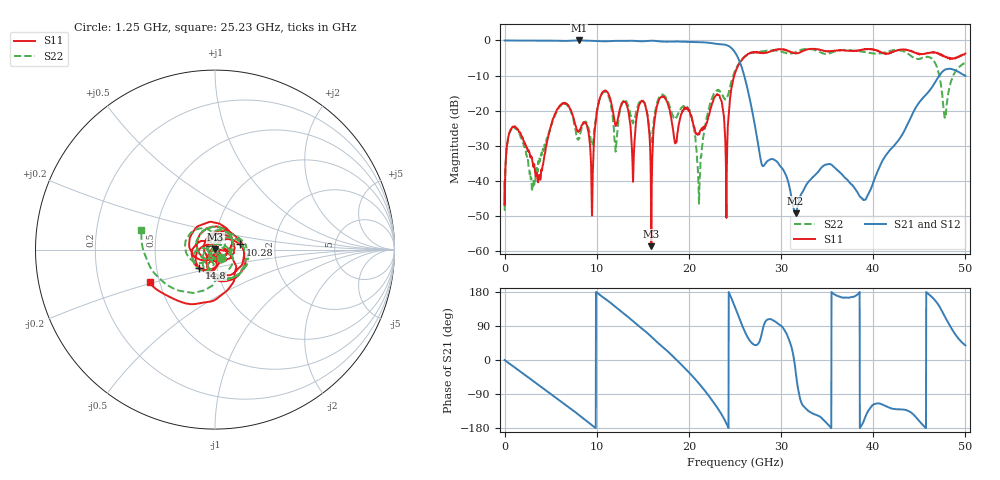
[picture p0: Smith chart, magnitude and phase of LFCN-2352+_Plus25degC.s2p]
! Mini-Circuits
! S2P DATA File Format
! Type: LOW PASS FILTER
! Model: LFCN-2352+
! All S Parameters are in dB deg format
! TEST CONDITIONS: INPUT POWER = 0 dBm - +25 deg C
# MHZ S DB R 50
!Frequency  S11 dB  S11 DEG  S21 dB  S21 DEG  S12 dB  S12 DEG  S22 dB  S22 DEG
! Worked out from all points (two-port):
!   2006 points, 10 MHz to 50 GHz, reference 50 ohm
!   highest |S21| = -0.01 dB at 8.075 GHz (marker M1); lowest = -49.1 dB at 31.57 GHz (marker M2)
!   |S21| within 3 dB of the highest: start of sweep to 24.9 GHz
!   lowest |S11| = -58.5 dB at 15.93 GHz (marker M3), VSWR 1.00, Z = 50.1 + j0.0787 ohm
!   |S11| at or under -10 dB: start of sweep to 24.93 GHz
!   |S22| runs from -48.2 to -2.4 dB; largest |S21 - S12| = 0.0027
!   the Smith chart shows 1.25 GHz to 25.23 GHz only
!   S11 on the Smith chart (normalised r, x): 1.25 GHz: 1.06, -0.10; 10.28 GHz: 1.32, +0.08; 14.8 GHz: 0.82, -0.17; 25.23 GHz: 0.44, -0.19
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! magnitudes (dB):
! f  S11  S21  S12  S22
! 10 MHz  -40.1  0.0  0.0  -40.3
! 1.25 GHz  -24.9  0.0  0.0  -25.2
! 3.1 GHz  -35.3  -0.1  -0.1  -42.0
! 6.1 GHz  -18.4  -0.1  -0.1  -18.5
! 8.075 GHz  -25.6  0.0  0.0  -27.7
! 8.35 GHz  -24.3  0.0  0.0  -25.3
! 9.5 GHz  -49.8  -0.1  -0.1  -29.8
! 10.28 GHz  -17.0  -0.2  -0.2  -17.1
! 13.95 GHz  -40.2  -0.1  -0.1  -23.6
! 14.8 GHz  -17.4  -0.2  -0.3  -17.0
! 15.93 GHz  -58.5  -0.1  -0.1  -28.8
! 16.68 GHz  -17.5  -0.2  -0.2  -16.8
! 21.12 GHz  -26.6  -0.5  -0.5  -43.9
! 23.12 GHz  -15.5  -1.0  -1.0  -14.3
! 24.07 GHz  -50.5  -1.3  -1.3  -16.6
! 25.02 GHz  -9.2  -3.5  -3.5  -8.5
! 25.23 GHz  -7.8  -4.4  -4.4  -7.4
! 31.57 GHz  -3.7  -49.1  -49.1  -3.3
! 33.35 GHz  -2.4  -39.1  -39.1  -2.6
! 41.67 GHz  -3.7  -31.6  -31.6  -3.1
! 47.8 GHz  -4.6  -8.3  -8.3  -21.2
! 50 GHz  -3.7  -10.1  -10.1  -6.3
